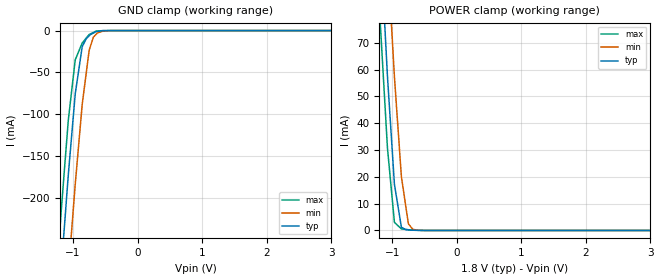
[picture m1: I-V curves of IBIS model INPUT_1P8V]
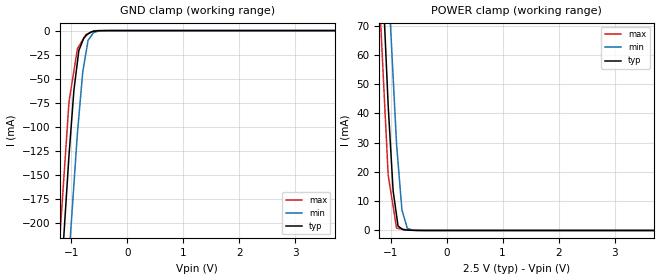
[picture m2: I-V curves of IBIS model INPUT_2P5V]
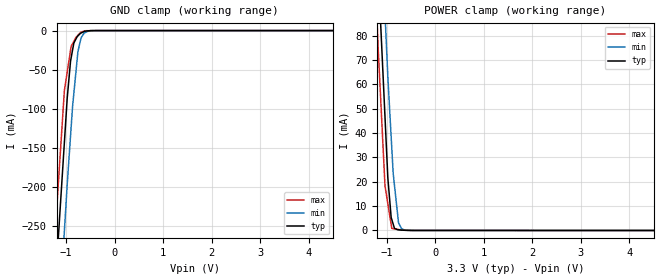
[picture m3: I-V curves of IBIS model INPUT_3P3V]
|IBIS File - Generated by SIMDE
|http://www.iometh.com/Product/SIMDE
[IBIS ver]   3.2
[File name]   sn75lvds83b.ibs
[File Rev]   1.2
[Date]   November 19, 2009, Monday
[Source]   TIspice Simulations at:
   Texas Instruments Incorporated.
   Analog-eLab, HPA
   12500 TI Blvd
   Dallas, TX -75243
   For Support e-mail: elab_ibis@list.ti.com
[Notes]   Revision History
   Rev 1.2: 11/19/2009
   - Added the ZQL package electrical model
   Rev 1.1: 11/06/2009
   - Resimulated to match the IV with measurement
   Rev 1.0: 11/02/2009
   - Initial model generated from TIspice simulations
[Disclaimer]
 This model is designed as an aid for customers of Texas Instruments.
 TI and its licensors and suppliers make no warranties, either expressed
 or implied, with respect to this  model, including the warranties of
 merchantability or fitness for a particular purpose.
 The model is provided solely on an "as is" basis. The entire risk as to
 its quality and performance is with the customer.
[Copyright] (C)Copyright 2009 Texas Instruments Incorporated.
   All rights reserved.
|   Component SN75LVDS83BDGG
[Component]   SN75LVDS83BDGG
[Manufacturer]  Texas Instruments Incorporated
[Package]   |56-pin DGG
| variable   typ   min   max
R_pkg   0.016676071   0.01202   0.02785
L_pkg   1.8464075n   1.32536n   3.11975n
C_pkg   0.597493393p   0.40408p   0.94255p
|-------------------------PIN------------------------------------------------
[Pin]  signal_name   model_name   R_pin   L_pin   C_pin
1   IOVCC   NC   0.02749   3.10562n  0.8865p
2   D5   INPUT   0.02553   2.77707n  0.93349p
3   D6   INPUT   0.02291   2.49299n  0.83295p
4   D7   INPUT   0.0204   2.22181n  0.73464p
5   GND   GND   0.01794   1.96679n  0.6051p
6   D8   INPUT   0.01476   1.65199n  0.5125p
7   D9   INPUT   0.0131   1.52892n  0.49376p
8   D10   INPUT   0.01401   1.59254n  0.54379p
9   VCC   NC   0.01383   1.55324n  0.52812p
10   D11   INPUT   0.01324   1.47155n  0.49738p
11   D12   INPUT   0.01296   1.42939n  0.48847p
12   D13   INPUT   0.01243   1.35656n  0.45645p
13   GND   GND   0.01224   1.34198n  0.44182p
14   D14   INPUT   0.01202   1.32536n  0.40408p
15   D15   INPUT   0.01202   1.32599n  0.40462p
16   D16   INPUT   0.01225   1.34214n  0.44189p
17   CLKSEL   INPUT   0.01243   1.35635n  0.45668p
18   D17   INPUT   0.01297   1.42997n  0.48849p
19   D18   INPUT   0.01324   1.47183n  0.49743p
20   D19   INPUT   0.01385   1.55426n  0.52797p
21   GND   GND   0.01402   1.59354n  0.54374p
22   D20   INPUT   0.01312   1.5301n   0.49346p
23   D21   INPUT   0.01492   1.66863n  0.51512p
24   D22   INPUT   0.01806   1.9806n   0.60737p
25   D23   INPUT   0.02041   2.22274n  0.73353p
26   IOVCC   NC   0.02291   2.49363n  0.83227p
27   D24   INPUT   0.02552   2.77657n  0.9331p
28   D25   INPUT   0.02747   3.09987n  0.88317p
29   GND   GND   0.02785   3.119n   0.89163p
30   D26   INPUT   0.02581   2.78543n  0.94255p
31   CLKIN   INPUT   0.02313   2.50065n  0.83854p
32   SHTDN   INPUT   0.02055   2.22807n  0.73579p
33   GND   GND   0.01802   1.97118n  0.60401p
34   PLLVCC   NC   0.01485   1.65956n  0.51275p
35   GND   GND   0.01311   1.52966n  0.49374p
36   GND   GND   0.01403   1.59356n  0.54394p
37   Y3P   DRIVER_p   0.01385   1.5544n   0.52814p
38   Y3M   DRIVER_n   0.01324   1.47176n  0.49763p
39   CLKOUTP   DRIVER_p   0.01297   1.42987n  0.48852p
40   CLKOUTM   DRIVER_n   0.01243   1.35645n  0.45656p
41   Y2P   DRIVER_p   0.01225   1.3422n   0.44171p
42   Y2M   DRIVER_n   0.01203   1.32756n  0.40506p
43   GND   GND   0.01205   1.32865n  0.40476p
44   LVDSVCC   NC   0.01225   1.34268n  0.44154p
45   Y1P   DRIVER_p   0.01244   1.35754n  0.45599p
46   Y1M   DRIVER_n   0.01298   1.43067n  0.48809p
47   Y0P   DRIVER_p   0.01326   1.47278n  0.49721p
48   Y0M   DRIVER_n   0.01385   1.55472n  0.5279p
49   GND   GND   0.01404   1.59438n  0.54349p
50   D27   INPUT   0.01311   1.53007n  0.49351p
51   D0   INPUT   0.01482   1.65929n  0.51274p
52   D1   INPUT   0.01799   1.96995n  0.60389p
53   GND   GND   0.02048   2.22593n  0.73461p
54   D2   INPUT   0.02301   2.49769n  0.83413p
55   D3   INPUT   0.02567   2.78334n  0.93545p
56   D4   INPUT   0.02774   3.11975n  0.88786p
|-------------------------DIFF PIN------------------------------------------
[Diff_pin]   inv_pin   vdiff   tdelay_typ   tdelay_min   tdelay_max
  37   38   NA   NA   NA   NA
  39   40   NA   NA   NA   NA
  41   42   NA   NA   NA   NA
  45   46   NA   NA   NA   NA
  47   48   NA   NA   NA   NA
[Model Selector]   INPUT
INPUT_1P8V   1.80V Input Model
INPUT_2P5V   2.50V Input Model
INPUT_3P3V   3.30V Input Model
|   Component SN75LVDS83BZQL
[Component]   SN75LVDS83BZQL
[Manufacturer]  Texas Instruments Incorporated
[Package]   |56-pin ZQL
| variable   typ   min   max
R_pkg   0.016676071   0.01202   0.02785
L_pkg   1.8464075n   1.32536n   3.11975n
C_pkg   0.597493393p   0.40408p   0.94255p
|-------------------------PIN------------------------------------------------
[Pin]  signal_name   model_name   R_pin   L_pin   C_pin
A1   GND   GND   0.15004   1.5913n   0.35319p
A2   CLKIN   INPUT   0.25173   1.8372n   0.33795p
A3   D26   INPUT   0.28461   1.9238n   0.28367p
A4   D24   INPUT   0.28925   1.9356n   0.33065p
A5   D23   INPUT   0.21972   1.6087n   0.30363p
A6   D22   INPUT   0.24592   1.8504n   0.25048p
B1   GND   GND   0.08038   1.0044n   0.42018p
B2   PLLVCC   NC   0.18735   1.5992n   0.46117p
B3   SHTDN   INPUT   0.25173   1.8372n   0.33795p
B4   D25   INPUT   0.32392   1.9784n   0.42988p
B5   D21   INPUT   0.29693   2.0045n   0.37944p
B6   D20   INPUT   0.24467   1.6511n   0.32995p
C1   Y3M   DRIVER_n   0.22788   1.5223n   0.32944p
C2   Y3P   DRIVER_p   0.28589   1.8404n   0.39517p
C3   GND   GND   0.2288   2.0067n   0.25159p
C4   IOVCC   NC   0.21611   1.6723n   0.53266p
C5   GND   GND   0.2288   2.0067n   0.25159p
C6   D19   INPUT   0.21563   1.3825n   0.30931p
D1   CLKM   DRIVER_n   0.19771   1.24n   0.27344p
D2   CLKP   DRIVER_p   0.25267   1.588n   0.35263p
D3   GND   GND   0.2288   2.0067n   0.25159p
D4   CLKSEL   INPUT   0.24971   1.6519n   0.40899p
D5   D18   INPUT   0.24054   1.4849n   0.36834p
D6   D17   INPUT   0.19172   1.1531n   0.27656p
E1   Y2M   DRIVER_n   0.17188   1.0474n   0.25747p
E2   Y2P   DRIVER_p   0.22426   1.3233n   0.322p
E3   NC   NC   0.2288   2.0067n   0.25159p
E4   NC   NC   0.2288   2.0067n   0.25159p
E5   D15   INPUT   0.20951   1.1892n   0.30765p
E6   D16   INPUT   0.17811   1.033n   0.24849p
F1   LVDSVCC   NC   0.1035   0.79109n  0.29462p
F2   GND   GND   0.2288   2.0067n   0.25159p
F3   NC   NC   0.2288   2.0067n   0.25159p
F4   NC   NC   0.2288   2.0067n   0.25159p
F5   GND   GND   0.2288   2.0067n   0.25159p
F6   D14   INPUT   0.1801   1.0583n   0.23934p
G1   Y1M   DRIVER_n   0.19341   1.1472n   0.27868p
G2   Y1P   DRIVER_p   0.22291   1.3036n   0.34043p
G3   GND   GND   0.2288   2.0067n   0.25159p
G4   IOVCC   NC   0.12021   0.9071n   0.53059p
G5   D12   INPUT   0.24857   1.5497n   0.35581p
G6   D13   INPUT   0.19802   1.2016n   0.2881p
H1   Y0M   DRIVER_n   0.21279   1.4079n   0.27946p
H2   Y0P   DRIVER_p   0.24183   1.6145n   0.36471p
H3   GND   GND   0.2288   2.0067n   0.25159p
H4   D10   INPUT   0.31922   2.0611n   0.51714p
H5   VCC   NC   0.18089   1.4677n   0.48501p
H6   D11   INPUT   0.22498   1.4533n   0.34349p
J1   D27   INPUT   0.18208   1.263n   0.24896p
J2   D0   INPUT   0.20929   1.2923n   0.34606p
J3   D3   INPUT   0.20418   1.243n   0.3888p
J4   D6   INPUT   0.20378   1.283n   0.33948p
J5   GND   GND   0.11663   1.0352n   0.38045p
J6   D9   INPUT   0.23538   1.5275n   0.30261p
K1   D1   INPUT   0.29843   2.129n   0.26949p
K2   D2   INPUT   0.22405   1.6701n   0.28076p
K3   D4   INPUT   0.27447   1.8488n   0.28023p
K4   D5   INPUT   0.28934   1.9446n   0.31693p
K5   D7   INPUT   0.29477   2.0184n   0.28661p
K6   D8   INPUT   0.23688   1.7704n   0.27179p
|-------------------------DIFF PIN------------------------------------------
[Diff_pin]   inv_pin   vdiff   tdelay_typ   tdelay_min   tdelay_max
  C2   C1   NA   NA   NA   NA
  D2   D1   NA   NA   NA   NA
  E2   E1   NA   NA   NA   NA
  G2   G1   NA   NA   NA   NA
  H2   H1   NA   NA   NA   NA
| Models and submodels in the file (5): INPUT_1P8V (Input), INPUT_2P5V (Input), INPUT_3P3V (Input), DRIVER_p (Output), DRIVER_n (Output)
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[Model]   INPUT_1P8V
Model_type   Input
Vinl = 0.6
Vinh = 1.2
|   typ   min   max
C_comp   0.250e-12   NA   NA
|C_comp (ON state)   1.000e-200   NA   NA
|C_comp (OFF state)   1.000e-200   NA   NA
[Voltage Range]   1.8   1.62   1.98
[Temperature Range]   25   125   -40
[Power Clamp Reference]   1.8   1.62   1.98
[GND Clamp Reference]   -0   -0   -0
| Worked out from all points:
|   GND clamp passes 1 mA (typ) near -0.61 V on its own axis
|   POWER clamp passes 1 mA (typ) near -0.84 V on its own axis
[GND Clamp]
|   Voltage   I(typ)   I(min)   I(max)
-1.8V     -975.1mA   -1.093A    -912.7mA
-1.29V    -400.9mA   -522.4mA   -331.6mA
-1.182V   -284.4mA   -405.6mA   -214.9mA
-1.074V   -173.3mA   -291.9mA   -107.7mA
-966.5mV  -75.82mA   -184mA     -35.05mA
-858.5mV  -19.2mA    -88.42mA   -14.94mA
-793.1mV  -9.35mA    -49.13mA   -8.758mA
-750.5mV  -6.265mA   -23.5mA    -4.726mA
-685.5mV  -2.945mA   -7.912mA   -2.209mA
-620.5mV  -1.074mA   -2.715mA   -436.7uA
-434.7mV  -14.42uA   -89.88uA   -6.122uA
3.6V      0A         0A         0A
[POWER Clamp]
|   Voltage   I(typ)   I(min)   I(max)
-1.8V     423mA      460.1mA    396.8mA
-1.182V   106.9mA    152.6mA    76.04mA
-1.074V   57.67mA    103.1mA    30.85mA
-966.5mV  17.25mA    57.37mA    3.035mA
-858.5mV  1.219mA    20.15mA    590.3uA
-793.1mV  328.8uA    9.478mA    403.9uA
-750.5mV  222.1uA    2.516mA    282.4uA
-685.5mV  116uA      506.8uA    164.4uA
-620.5mV  56.7uA     124.1uA    71.72uA
3.6V      0A         0A         0A
[Model]   INPUT_2P5V
Model_type   Input
Vinl = 0.85
Vinh = 1.65
|   typ   min   max
C_comp   0.250e-12   NA   NA
|C_comp (ON state)   1.000e-200   NA   NA
|C_comp (OFF state)   1.000e-200   NA   NA
[Voltage Range]   2.5   2.25   2.75
[Temperature Range]   25   125   -40
[Power Clamp Reference]   2.5   2.25   2.75
[GND Clamp Reference]   -0   -0   -0
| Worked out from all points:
|   GND clamp passes 1 mA (typ) near -0.62 V on its own axis
|   POWER clamp passes 1 mA (typ) near -0.83 V on its own axis
[GND Clamp]
|   Voltage   I(typ)   I(min)   I(max)
-2.5V     -1.598A    -1.7A      -1.549A
-1.342V   -412.5mA   -522mA     -350.1mA
-1.192V   -266.6mA   -376mA     -203.8mA
-1.042V   -130mA     -235.3mA   -74.28mA
-954.2mV  -62.05mA   -160mA     -41.81mA
-892.3mV  -32.95mA   -107.2mA   -19.01mA
-866mV    -20.6mA    -89.62mA   -16.41mA
-796.7mV  -10.65mA   -43.16mA   -9.546mA
-701.1mV  -3.441mA   -10.13mA   -3.058mA
-638.4mV  -1.19mA    -4.876mA   -1.374mA
-414.2mV  -27.81uA   -59.45uA   -6.296uA
5V        0A         0A         0A
[POWER Clamp]
|   Voltage   I(typ)   I(min)   I(max)
-2.5V     762.8mA    787.5mA    743.7mA
-1.192V   107.2mA    150.6mA    77.11mA
-1.042V   42.8mA     85.55mA    18.91mA
-954.2mV  13.59mA    52.58mA    8.265mA
-892.3mV  5.111mA    29.43mA    791.8uA
-866mV    1.512mA    23.28mA    704.4uA
-796.7mV  547.7uA    7.043mA    473.5uA
-701.1mV  142.3uA    743.6uA    226.3uA
-605.4mV  55.04uA    97.36uA    72.76uA
5V        0A         0A         0A
[Model]   INPUT_3P3V
Model_type   Input
Vinl = 1.15
Vinh = 2.15
|   typ   min   max
C_comp   0.250e-12   NA   NA
|C_comp (ON state)   1.000e-200   NA   NA
|C_comp (OFF state)   1.000e-200   NA   NA
[Voltage Range]   3.3   3   3.6
[Temperature Range]   25   125   -40
[Power Clamp Reference]   3.3   3   3.6
[GND Clamp Reference]   -0   -0   -0
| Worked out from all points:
|   GND clamp passes 1 mA (typ) near -0.62 V on its own axis
|   POWER clamp passes 1 mA (typ) near -0.84 V on its own axis
[GND Clamp]
|   Voltage   I(typ)   I(min)   I(max)
-3.3V     -2.716A    -2.824A    -2.674A
-1.376V   -495.1mA   -616.3mA   -426.6mA
-1.178V   -279.5mA   -400.6mA   -210mA
-1.038V   -143.6mA   -257.1mA   -76.99mA
-979.8mV  -86.53mA   -196.9mA   -53.17mA
-911.3mV  -39.21mA   -135mA     -25.27mA
-842.8mV  -15.86mA   -80.22mA   -13.7mA
-759.5mV  -6.816mA   -27.06mA   -6.007mA
-701.9mV  -3.378mA   -11.27mA   -2.095mA
-629.3mV  -1.17mA    -3.134mA   -691.6uA
-474.1mV  -38.94uA   -199.7uA   -10.81uA
6.6V      0A         0A         0A
[POWER Clamp]
|   Voltage   I(typ)   I(min)   I(max)
-3.3V     1.253A     1.262A     1.236A
-1.376V   204.6mA    247.1mA    173.4mA
-1.178V   106.3mA    151.3mA    74.25mA
-1.038V   46.62mA    89.18mA    18.31mA
-979.8mV  21.59mA    63.12mA    11mA
-911.3mV  5.367mA    38.44mA    2.44mA
-898.9mV  4.549mA    33.96mA    887.7uA
-869.7mV  2.626mA    23.44mA    768.3uA
-842.8mV  855.4uA    18.48mA    658.3uA
-759.5mV  263.8uA    3.144mA    380.9uA
-629.3mV  77.77uA    157.4uA    119.6uA
6.6V      0A         0A         0A
